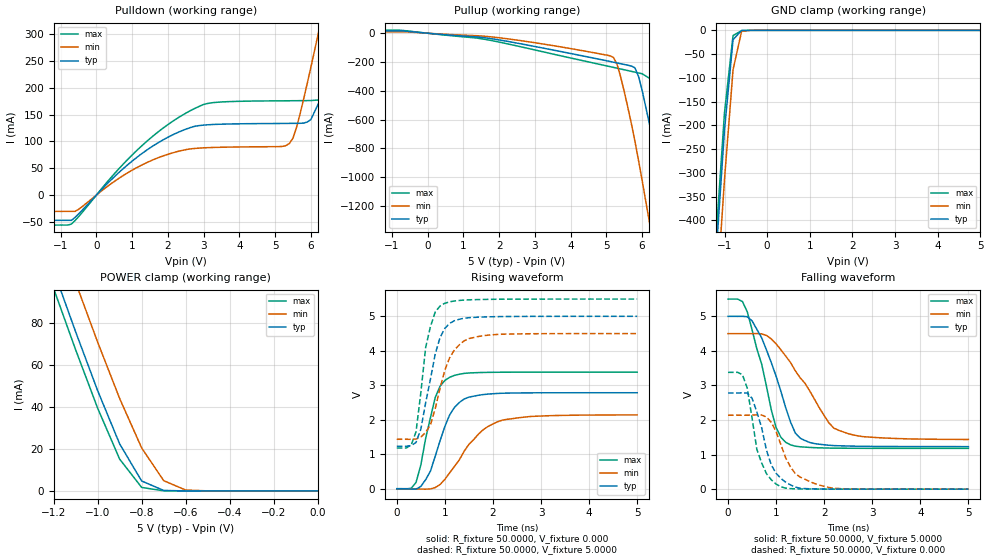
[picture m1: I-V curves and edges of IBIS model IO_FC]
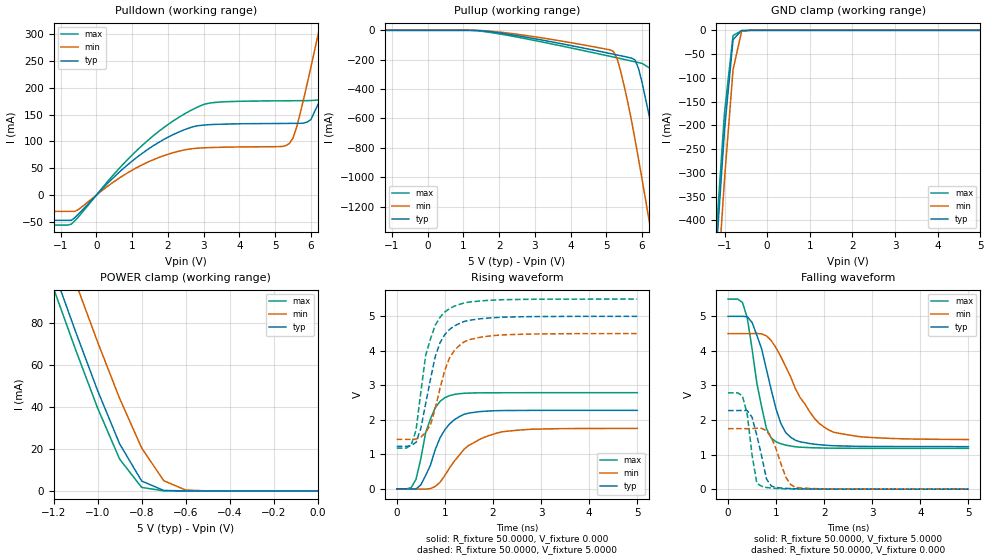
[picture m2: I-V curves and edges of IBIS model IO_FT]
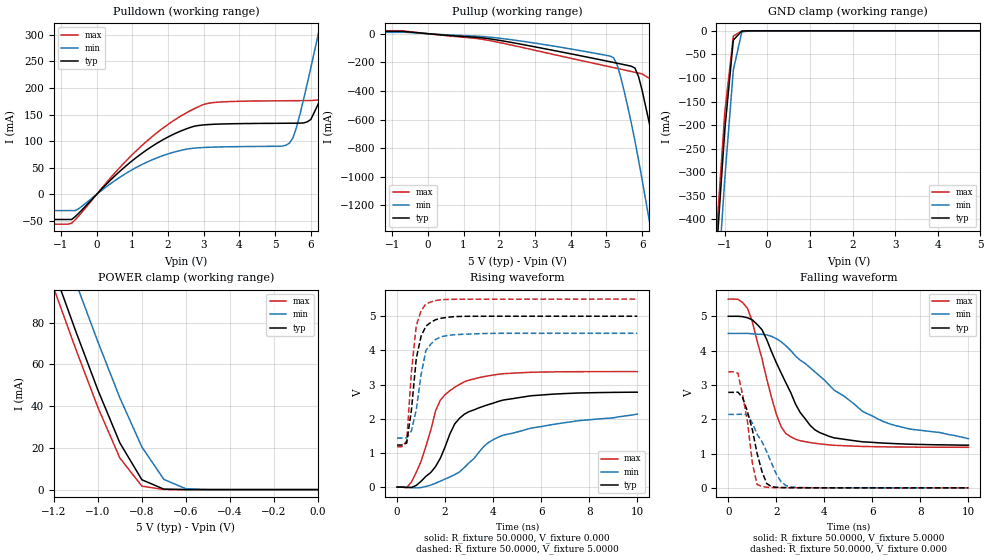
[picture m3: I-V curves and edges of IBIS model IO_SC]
| Xilinx XC4KE IBIS file
[IBIS ver]   2.1
[File name]   xc4ke.ibs
[File Rev]   2.4
[Date]   Aug 21, 2002
[Source]   Hspice simulations (05-1t: TT, SS, FF)
[Notes]   Xilinx IBIS model for XC4KE I/O
   The package models are provided for HQ208, PQ100, PQ160,
   PQ208, and TQ144 package types, with HQ208 being selected
   as a default. Please make your own selection of the packages
   by commenting out the unused ones.
   COMMENTS: Models include process corners for MIN and MAX.
[Disclaimer] The data in this model is derived from SPICE simulations using
   modeling information extracted from the target process. While
   a great deal of care has been taken to provide information
   that is accurate, this model is considered preliminary as it
   has not been verified by actual silicon measurement. Treat the
   data in this model as preliminary until actual silicon
   verification is performed.
[Copyright]   Copyright 1998, Xilinx Inc., All rights reserved
|   Component XC4KE
|   >>> Make Your Selection of the Package type Below <<<
[Component]   XC4KE
[Manufacturer]   Xilinx Inc.
[Package]
| For package type HQ208:
| variable   typ   min   max
R_pkg   0.160   0.120   0.200
L_pkg   11.00nH   6.40nH   15.70nH
C_pkg   1.70pF   1.00pF   2.40pF
| For package type PQ100:
| variable   typ   min   max
|R_pkg   0.084   0.07   0.098
|L_pkg   7.90nH   3.70nH   12.10nH
|C_pkg   1.10pF   0.65pF   1.50pF
| For package type PQ160:
| variable   typ   min   max
|R_pkg   0.183   0.159   0.207
|L_pkg   17.35nH   9.10nH   25.60nH
|C_pkg   1.85pF   1.00pF   2.70pF
| For package type PQ208:
| variable   typ   min   max
|R_pkg   0.150   0.132   0.169
|L_pkg   16.7nH   9.10nH   24.20nH
|C_pkg   1.90pF   1.00pF   2.80pF
| For package type TQ144:
| variable   typ   min   max
|R_pkg   0.150   0.111   0.137
|L_pkg   16.7nH   6.8nH   9.2nH
|C_pkg   1.90pF   0.70pF   1.30pF
| Note: The following pin list specifies all the models that are provided
|   in this ibis file.
|   The pin name is arbitrarily numbered and does not corresponds
|   to the pinout in the product package. Add the device pinout to
|   match the package type and the pinout for the particular design.
|   The model_name is explained as follows:
|   IO_FC: Fast slew rate, CMOS compatible
|   IO_FT: Fast slew rate, TTL compatible
|   IO_SC: Slow slew rate, CMOS compatible
|   IO_ST: Slow slew rate, TTL compatible
|   Please select the models accordingly.
[Pin]  signal_name   model_name   R_pin   L_pin   C_pin
IO1   IO_FC   IO_FC
IO2   IO_FT   IO_FT
IO3   IO_SC   IO_SC
IO4   IO_ST   IO_ST
PGND   GND   GND
VCCO   VDD   POWER
| Models and submodels in the file (4): IO_FC (I/O), IO_FT (I/O), IO_SC (I/O), IO_ST (I/O)
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|   Model IO_FC
[Model]   IO_FC
Model_type   I/O
Polarity   Non-Inverting
Enable   Active-Low
Vinh  = 2.0V
Vinl  = 0.8V
Vmeas =   2.5000V
Cref =  50.0000pF
Rref =   1.0000M
Vref =  0.000V
C_comp   8.00pF   6.00pF   10.00pF
[Temperature Range]   27.0000   100.0000   0.000
[Voltage Range]   5.0000V   4.5000V   5.5000V
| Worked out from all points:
|   slope of the pulldown table from 0 to 0.75 V, typ, clamps not added: 15.2 ohm
|   slope of the pullup table from 0 to 0.75 V, typ, clamps not added: 49.2 ohm
|   GND clamp passes 1 mA (typ) near -0.61 V on its own axis
|   POWER clamp passes 1 mA (typ) near -0.72 V on its own axis
|   rising waveform, R_fixture 50.0000, V_fixture 0.000: 20-80 % time 428ps typ, 716ps min, 319ps max; typ from 0 V to 2.78 V
|   rising waveform, R_fixture 50.0000, V_fixture 5.0000: 20-80 % time 337ps typ, 397ps min, 254ps max; typ from 1.23 V to 5 V
|   falling waveform, R_fixture 50.0000, V_fixture 5.0000: 20-80 % time 552ps typ, 857ps min, 453ps max; typ from 5 V to 1.23 V
|   falling waveform, R_fixture 50.0000, V_fixture 0.000: 20-80 % time 358ps typ, 440ps min, 301ps max; typ from 2.78 V to 0 V
[Pulldown]
| voltage   I(typ)   I(min)   I(max)
-5V       -47.22mA   -30.5mA    -56mA
-700mV    -47.22mA   -30.5mA    -54.14mA
1V        63.37mA    46.41mA    74.73mA
2.5V      122.8mA    84.67mA    152.7mA
5.3V      133.6mA    92.17mA    175.9mA
5.6V      133.8mA    126.2mA    176mA
6V        140.7mA    238mA      176.3mA
6.4V      196.9mA    359.3mA    178.3mA
6.8V      314.8mA    483mA      199.9mA
7.2V      438.1mA    607.8mA    286.2mA
7.6V      562.9mA    733.1mA    407.7mA
10V       1.321A     1.49A      1.163A
[Pullup]
| voltage   I(typ)   I(min)   I(max)
-5V       15.71mA    9.538mA    20.91mA
-700mV    15.71mA    9.538mA    19.58mA
1.6V      -31.59mA   -21.12mA   -42.31mA
5.1V      -196mA     -156.5mA   -231.7mA
5.3V      -206.3mA   -215.4mA   -242.6mA
5.8V      -240.2mA   -749.4mA   -270.1mA
6V        -394.4mA   -1.019A    -281.2mA
6.4V      -849.1mA   -1.586A    -341.6mA
6.8V      -1.353A    -2.164A    -771.1mA
7.2V      -1.924A    -2.748A    -1.249A
7.6V      -2.506A    -3.334A    -1.758A
10V       -6.046A    -6.875A    -5.275A
[GND_clamp]
| voltage   I(typ)   I(min)   I(max)
-5V       -6.041A    -6.132A    -6.009A
-1.2V     -475.4mA   -581.5mA   -437mA
-1V       -209.6mA   -313.5mA   -172.9mA
-800mV    -19.58mA   -83.01mA   -10.94mA
-600mV    -371.5uA   -2.252mA   -681.5uA
-400mV    -2.131uA   -13.41uA   -2.859uA
5V        208pA      25.02uA    188.3pA
[POWER_clamp]
| voltage   I(typ)   I(min)   I(max)
-5V       1.297A     1.316A     1.29A
-1.2V     105mA      128.5mA    96.44mA
-1.1V     75.81mA    99.25mA    67.26mA
-1V       47.76mA    70.87mA    39.43mA
-900mV    22.39mA    43.99mA    15.14mA
-800mV    4.715mA    20.43mA    1.664mA
-700mV    224.2uA    4.878mA    49.53uA
-600mV    6.639uA    413.1uA    1.44uA
-500mV    218.8nA    25.05uA    69.52nA
0V        208pA      392.6pA    227.8pA
[Ramp]
| variable   typ   min   max
dV/dt_r   1.6698/0.4244n   1.2840/0.7154n   2.0280/0.2848n
dV/dt_f   2.2614/0.5496n   1.8372/0.8608n   2.5914/0.4217n
R_load = 50.0000
[Rising Waveform]
R_fixture = 50.0000
V_fixture = 0.000
| time   V(typ)   V(min)   V(max)
0s        0V         0V         0V
400ps     -11.43mV   -4.58mV    180.8mV
500ps     65.57mV    -9.967mV   684.8mV
600ps     262.3mV    -12.78mV   1.456V
800ps     944.7mV    34.3mV     2.648V
1.1ns     2.14V      459.7mV    3.232V
1.4ns     2.602V     1.084V     3.343V
1.7ns     2.711V     1.587V     3.368V
2.2ns     2.769V     1.991V     3.378V
5ns       2.783V     2.14V      3.38V
[Rising Waveform]
R_fixture = 50.0000
V_fixture = 5.0000
V_fixture_min = 4.5000
V_fixture_max = 5.5000
| time   V(typ)   V(min)   V(max)
0s        1.231V     1.434V     1.181V
300ps     1.253V     1.432V     1.271V
400ps     1.341V     1.441V     1.648V
500ps     1.725V     1.497V     2.781V
600ps     2.484V     1.632V     4.09V
800ps     3.91V      2.325V     5.126V
900ps     4.383V     2.914V     5.297V
1.1ns     4.795V     3.8V       5.419V
1.5ns     4.959V     4.353V     5.477V
5ns       4.999V     4.499V     5.499V
[Falling Waveform]
R_fixture = 50.0000
V_fixture = 5.0000
V_fixture_min = 4.5000
V_fixture_max = 5.5000
| time   V(typ)   V(min)   V(max)
0s        5V         4.5V       5.5V
300ps     5.001V     4.499V     5.43V
400ps     4.99V      4.5V       5.134V
700ps     4.38V      4.494V     3.62V
1ns       3.271V     4.204V     1.784V
1.2ns     2.357V     3.85V      1.356V
1.5ns     1.476V     3.224V     1.226V
2.1ns     1.271V     1.916V     1.189V
2.3ns     1.256V     1.704V     1.186V
5ns       1.231V     1.438V     1.181V
[Falling Waveform]
R_fixture = 50.0000
V_fixture = 0.000
| time   V(typ)   V(min)   V(max)
0s        2.783V     2.141V     3.38V
300ps     2.786V     2.14V      3.311V
500ps     2.631V     2.143V     2.058V
600ps     2.236V     2.151V     1.151V
700ps     1.778V     2.146V     757.1mV
900ps     700.3mV    1.933V     270.3mV
1.1ns     309.6mV    1.288V     69.53mV
1.4ns     59.05mV    450.5mV    10.52mV
2.1ns     3.875mV    49.18mV    1.965mV
5ns       174.4uV    326.9uV    145.7uV
|   Model IO_FT
[Model]   IO_FT
Model_type   I/O
Polarity   Non-Inverting
Enable   Active-Low
Vinh  = 2.0V
Vinl  = 0.8V
Vmeas =   2.5000V
Cref =  50.0000pF
Rref =   1.0000M
Vref =  0.000V
C_comp   8.00pF   6.00pF   10.00pF
[Temperature Range]   27.0000   100.0000   0.000
[Voltage Range]   5.0000V   4.5000V   5.5000V
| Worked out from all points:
|   slope of the pulldown table from 0 to 0.75 V, typ, clamps not added: 15.2 ohm
|   GND clamp passes 1 mA (typ) near -0.61 V on its own axis
|   POWER clamp passes 1 mA (typ) near -0.72 V on its own axis
|   rising waveform, R_fixture 50.0000, V_fixture 0.000: 20-80 % time 438ps typ, 700ps min, 315ps max; typ from 0 V to 2.27 V
|   rising waveform, R_fixture 50.0000, V_fixture 5.0000: 20-80 % time 371ps typ, 400ps min, 341ps max; typ from 1.23 V to 5 V
|   falling waveform, R_fixture 50.0000, V_fixture 5.0000: 20-80 % time 427ps typ, 720ps min, 317ps max; typ from 5 V to 1.23 V
|   falling waveform, R_fixture 50.0000, V_fixture 0.000: 20-80 % time 226ps typ, 272ps min, 164ps max; typ from 2.27 V to 0 V
[Pulldown]
| voltage   I(typ)   I(min)   I(max)
-5V       -47.22mA   -30.5mA    -56mA
-700mV    -47.22mA   -30.5mA    -54.14mA
1V        63.37mA    46.41mA    74.73mA
2.5V      122.8mA    84.67mA    152.7mA
5.3V      133.6mA    92.17mA    175.9mA
5.6V      133.8mA    126.2mA    176mA
6V        140.7mA    238mA      176.3mA
6.4V      196.9mA    359.3mA    178.3mA
6.8V      314.8mA    483mA      199.9mA
7.2V      438.1mA    607.8mA    286.2mA
7.6V      562.9mA    733.1mA    407.7mA
10V       1.321A     1.49A      1.163A
[Pullup]
| voltage   I(typ)   I(min)   I(max)
-5V       200pA      348.8pA    219.9pA
1.3V      -437uA     -213.6uA   -1.434mA
5.1V      -157.5mA   -132.9mA   -176.7mA
5.3V      -167.7mA   -191.5mA   -187.3mA
5.4V      -172.8mA   -277.5mA   -192.7mA
5.8V      -201mA     -739.2mA   -214.2mA
6V        -354.6mA   -1.014A    -225.1mA
6.4V      -808.8mA   -1.583A    -285.1mA
6.8V      -1.343A    -2.162A    -713.3mA
7.2V      -1.919A    -2.746A    -1.192A
7.6V      -2.503A    -3.332A    -1.744A
10V       -6.043A    -6.873A    -5.271A
[GND_clamp]
| voltage   I(typ)   I(min)   I(max)
-5V       -6.041A    -6.132A    -6.009A
-1.2V     -475.4mA   -581.5mA   -437mA
-1V       -209.6mA   -313.5mA   -172.9mA
-800mV    -19.58mA   -83.01mA   -10.94mA
-600mV    -371.5uA   -2.252mA   -681.5uA
-400mV    -2.131uA   -13.41uA   -2.859uA
5V        208pA      25.02uA    188.3pA
[POWER_clamp]
| voltage   I(typ)   I(min)   I(max)
-5V       1.297A     1.316A     1.29A
-1.2V     105mA      128.5mA    96.44mA
-1.1V     75.81mA    99.25mA    67.26mA
-1V       47.76mA    70.87mA    39.43mA
-900mV    22.39mA    43.99mA    15.14mA
-800mV    4.715mA    20.43mA    1.664mA
-700mV    224.2uA    4.878mA    49.53uA
-600mV    6.639uA    413.1uA    1.44uA
-500mV    218.8nA    25.05uA    69.52nA
0V        208pA      392.6pA    227.8pA
[Ramp]
| variable   typ   min   max
dV/dt_r   1.3644/0.4128n   1.0500/0.6960n   1.6716/0.2753n
dV/dt_f   2.2614/0.4102n   1.8378/0.7181n   2.5914/0.2787n
R_load = 50.0000
[Rising Waveform]
R_fixture = 50.0000
V_fixture = 0.000
| time   V(typ)   V(min)   V(max)
0s        0V         0V         0V
300ps     -7.966mV   -660.8uV   36.59mV
400ps     -5.38mV    -4.572mV   276.9mV
500ps     115.8mV    -9.685mV   870.5mV
600ps     383.6mV    -8.893mV   1.626V
800ps     1.139V     69.08mV    2.352V
1.1ns     1.884V     612.1mV    2.702V
1.5ns     2.195V     1.262V     2.775V
2.2ns     2.268V     1.655V     2.785V
5ns       2.274V     1.75V      2.786V
[Rising Waveform]
R_fixture = 50.0000
V_fixture = 5.0000
V_fixture_min = 4.5000
V_fixture_max = 5.5000
| time   V(typ)   V(min)   V(max)
0s        1.231V     1.434V     1.181V
300ps     1.253V     1.432V     1.274V
400ps     1.348V     1.441V     1.692V
500ps     1.748V     1.498V     2.794V
600ps     2.465V     1.633V     3.862V
800ps     3.833V     2.328V     4.742V
1.1ns     4.623V     3.799V     5.226V
1.4ns     4.849V     4.259V     5.385V
1.9ns     4.949V     4.424V     5.46V
5ns       4.999V     4.499V     5.499V
[Falling Waveform]
R_fixture = 50.0000
V_fixture = 5.0000
V_fixture_min = 4.5000
V_fixture_max = 5.5000
| time   V(typ)   V(min)   V(max)
0s        5V         4.5V       5.5V
300ps     5.002V     4.499V     5.404V
400ps     4.988V     4.5V       4.962V
500ps     4.826V     4.501V     4.064V
800ps     3.462V     4.434V     1.75V
1ns       2.318V     4.088V     1.371V
1.3ns     1.505V     3.26V      1.25V
1.7ns     1.321V     2.236V     1.202V
2.1ns     1.264V     1.709V     1.188V
5ns       1.231V     1.437V     1.181V
[Falling Waveform]
R_fixture = 50.0000
V_fixture = 0.000
| time   V(typ)   V(min)   V(max)
0s        2.274V     1.75V      2.786V
300ps     2.278V     1.75V      2.698V
400ps     2.275V     1.75V      2.171V
600ps     1.553V     1.764V     170.3mV
700ps     958.8mV    1.759V     83.71mV
800ps     295.3mV    1.69V      48.98mV
900ps     92.41mV    1.498V     32.77mV
1.2ns     23.46mV    353.7mV    11.45mV
1.4ns     12.15mV    55.6mV     6.06mV
5ns       153.6uV    290.8uV    121uV
|   Model IO_SC
[Model]   IO_SC
Model_type   I/O
Polarity   Non-Inverting
Enable   Active-Low
Vinh  = 2.0V
Vinl  = 0.8V
Vmeas =   2.5000V
Cref =  50.0000pF
Rref =   1.0000M
Vref =  0.000V
C_comp   8.00pF   6.00pF   10.00pF
[Temperature Range]   27.0000   100.0000   0.000
[Voltage Range]   5.0000V   4.5000V   5.5000V
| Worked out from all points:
|   slope of the pulldown table from 0 to 0.75 V, typ, clamps not added: 15.2 ohm
|   slope of the pullup table from 0 to 0.75 V, typ, clamps not added: 49.2 ohm
|   GND clamp passes 1 mA (typ) near -0.61 V on its own axis
|   POWER clamp passes 1 mA (typ) near -0.72 V on its own axis
|   rising waveform, R_fixture 50.0000, V_fixture 0.000: 20-80 % time 1.5ns typ, 2.93ns min, 1.05ns max; typ from 0 V to 2.78 V
|   rising waveform, R_fixture 50.0000, V_fixture 5.0000: 20-80 % time 406ps typ, 439ps min, 319ps max; typ from 1.23 V to 5 V
|   falling waveform, R_fixture 50.0000, V_fixture 5.0000: 20-80 % time 1.58ns typ, 3.39ns min, 982ps max; typ from 5 V to 1.24 V
|   falling waveform, R_fixture 50.0000, V_fixture 0.000: 20-80 % time 575ps typ, 874ps min, 421ps max; typ from 2.78 V to 0 V
[Pulldown]
| voltage   I(typ)   I(min)   I(max)
-5V       -47.22mA   -30.5mA    -56mA
-700mV    -47.22mA   -30.5mA    -54.14mA
1V        63.37mA    46.41mA    74.73mA
2.5V      122.8mA    84.67mA    152.7mA
5.3V      133.6mA    92.17mA    175.9mA
5.6V      133.8mA    126.2mA    176mA
6V        140.7mA    238mA      176.3mA
6.4V      196.9mA    359.3mA    178.3mA
6.8V      314.8mA    483mA      199.9mA
7.2V      438.1mA    607.8mA    286.2mA
7.6V      562.9mA    733.1mA    407.7mA
10V       1.321A     1.49A      1.163A
[Pullup]
| voltage   I(typ)   I(min)   I(max)
-5V       15.71mA    9.538mA    20.91mA
-700mV    15.71mA    9.538mA    19.58mA
1.6V      -31.59mA   -21.12mA   -42.31mA
5.1V      -196mA     -156.5mA   -231.7mA
5.3V      -206.3mA   -215.4mA   -242.6mA
5.8V      -240.2mA   -749.4mA   -270.1mA
6V        -394.4mA   -1.019A    -281.2mA
6.4V      -849.1mA   -1.586A    -341.6mA
6.8V      -1.353A    -2.164A    -771.1mA
7.2V      -1.924A    -2.748A    -1.249A
7.6V      -2.506A    -3.334A    -1.758A
10V       -6.046A    -6.875A    -5.275A
[GND_clamp]
| voltage   I(typ)   I(min)   I(max)
-5V       -6.041A    -6.132A    -6.009A
-1.2V     -475.4mA   -581.5mA   -437mA
-1V       -209.6mA   -313.5mA   -172.9mA
-800mV    -19.58mA   -83.01mA   -10.94mA
-600mV    -371.5uA   -2.252mA   -681.5uA
-400mV    -2.131uA   -13.41uA   -2.859uA
5V        208pA      25.02uA    188.3pA
[POWER_clamp]
| voltage   I(typ)   I(min)   I(max)
-5V       1.297A     1.316A     1.29A
-1.2V     105mA      128.5mA    96.44mA
-1.1V     75.81mA    99.25mA    67.26mA
-1V       47.76mA    70.87mA    39.43mA
-900mV    22.39mA    43.99mA    15.14mA
-800mV    4.715mA    20.43mA    1.664mA
-700mV    224.2uA    4.878mA    49.53uA
-600mV    6.639uA    413.1uA    1.44uA
-500mV    218.8nA    25.05uA    69.52nA
0V        208pA      392.6pA    227.8pA
[Ramp]
| variable   typ   min   max
dV/dt_r   1.6662/1.5244n   1.2390/2.6876n   2.0280/0.9895n
dV/dt_f   2.2536/1.5802n   1.7694/3.1511n   2.5908/0.9151n
R_load = 50.0000
[Rising Waveform]
R_fixture = 50.0000
V_fixture = 0.000
| time   V(typ)   V(min)   V(max)
0s        0V         0V         0V
600ps     -11.41mV   -13.74mV   148.5mV
1ns       170.7mV    -12.88mV   756.7mV
1.4ns     424.9mV    57.49mV    1.656V
1.8ns     841.4mV    171.9mV    2.541V
2.4ns     1.847V     363.8mV    2.92V
2.8ns     2.132V     572.9mV    3.081V
3.8ns     2.413V     1.304V     3.256V
4.4ns     2.544V     1.515V     3.317V
10ns      2.777V     2.135V     3.38V
[Rising Waveform]
R_fixture = 50.0000
V_fixture = 5.0000
V_fixture_min = 4.5000
V_fixture_max = 5.5000
| time   V(typ)   V(min)   V(max)
0s        1.231V     1.434V     1.181V
200ps     1.23V      1.434V     1.181V
400ps     1.286V     1.438V     1.349V
600ps     2.267V     1.649V     3.39V
800ps     3.763V     2.265V     4.725V
1ns       4.415V     3.29V      5.156V
1.2ns     4.707V     3.999V     5.361V
1.6ns     4.896V     4.318V     5.457V
2.4ns     4.989V     4.458V     5.495V
10ns      4.999V     4.5V       5.5V
[Falling Waveform]
R_fixture = 50.0000
V_fixture = 5.0000
V_fixture_min = 4.5000
V_fixture_max = 5.5000
| time   V(typ)   V(min)   V(max)
0s        5V         4.5V       5.5V
800ps     4.957V     4.501V     5.232V
1.4ns     4.612V     4.474V     3.773V
2ns       3.647V     4.348V     2.149V
2.2ns     3.349V     4.259V     1.782V
2.6ns     2.778V     4.002V     1.49V
3.4ns     1.827V     3.506V     1.321V
4.4ns     1.458V     2.852V     1.24V
6.6ns     1.3V       1.893V     1.194V
10ns      1.244V     1.431V     1.182V
[Falling Waveform]
R_fixture = 50.0000
V_fixture = 0.000
| time   V(typ)   V(min)   V(max)
0s        2.783V     2.141V     3.38V
400ps     2.789V     2.141V     3.341V
600ps     2.623V     2.148V     2.695V
800ps     2.219V     2.135V     1.924V
1ns       1.702V     1.89V      734.4mV
1.2ns     1.003V     1.563V     98.78mV
1.6ns     125.5mV    1.055V     19.5mV
2.2ns     10.54mV    176.6mV    5.117mV
2.6ns     5.293mV    28.86mV    3.37mV
10ns      82.53uV    436.6uV    25.98uV
